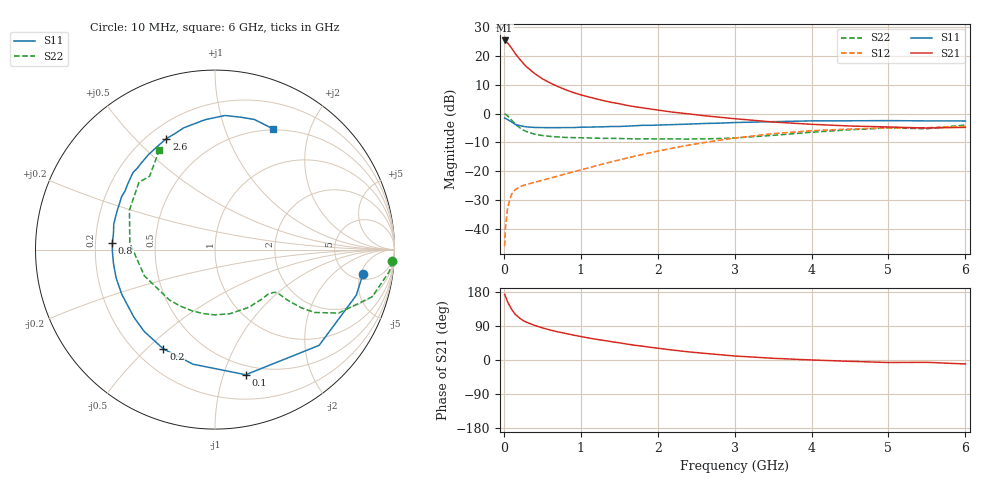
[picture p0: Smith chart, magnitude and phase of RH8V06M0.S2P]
! SIEMENS Small Signal Semiconductors
! BFR106
! Si NPN RF Bipolar Junction Transistor in SOT23
! VCE = 8 V  IC = 6 mA
! Common Emitter S-Parameters:  August  1996
# GHz  S  MA  R  50
!  f  S11  S21  S12  S22
! GHz  MAG  ANG  MAG  ANG  MAG  ANG  MAG  ANG
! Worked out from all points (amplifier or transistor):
!   36 points, 10 MHz to 6 GHz, reference 50 ohm
!   highest |S21| = 25.4 dB at 10 MHz (marker M1)
!   |S21| within 3 dB of that: start of sweep to 109.4 MHz
!   unconditionally stable (mu >= 1): 589.9 MHz to 1.841 GHz; 5.092 GHz to end of sweep
!   at 250 MHz: K = 0.55, MSG = 21.2 dB, |S12| = -24.9 dB
!   at 1.4 GHz: K = 1.11, MAG = 8.3 dB, |S12| = -16.7 dB
!   at 6 GHz: K = 1.01, MAG = -0.9 dB, |S12| = -4.4 dB
!   S11 on the Smith chart (normalised r, x): 10 MHz: 6.22, -5.51; 100 MHz: 0.41, -1.19; 200 MHz: 0.31, -0.56; 800 MHz: 0.27, +0.03; 2.6 GHz: 0.27, +0.62; 6 GHz: 0.49, +1.48
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0.01  0.8357 -9.2  18.66 173.5  0.005 88.2  0.9907 -3.8
0.02  0.8275 -17.9  18.42 168.7  0.0101 82.7  0.9778 -7.3
0.05  0.7881 -42.6  16.81 152.9  0.0239 68.8  0.9142 -16.7
0.1  0.7179 -76.2  13.79 134.0  0.0398 55.2  0.7738 -27.2
0.15  0.6501 -100.9  10.98 120.0  0.0479 47.3  0.6555 -32.3
0.2  0.6234 -117.5  9.019 111.4  0.0531 44.1  0.5785 -34.0
0.25  0.6031 -130.8  7.531 104.1  0.0566 42.1  0.5209 -34.6
0.3  0.5883 -140.2  6.429 99.2  0.0592 42.4  0.4853 -34.9
0.4  0.5761 -154.5  4.98 91.4  0.0641 43.9  0.4402 -34.7
0.5  0.5729 -164.2  4.036 84.8  0.0697 46.4  0.417 -35.0
0.6  0.5709 -172.1  3.42 79.3  0.0756 49.2  0.4031 -36.3
0.8  0.5733 176.3  2.61 70.2  0.0897 54.7  0.3863 -40.1
0.9  0.5727 171.1  2.33 65.9  0.0972 57.2  0.3833 -42.1
1.1  0.5838 161.4  1.952 58.2  0.1143 60.6  0.3783 -48.1
1.6  0.6073 143.5  1.392 42.0  0.1692 64.6  0.3678 -64.9
2.2  0.6456 125.2  1.06 26.1  0.253 61.8  0.3634 -90.3
2.6  0.6746 113.7  0.922 17.7  0.314 56.7  0.3642 -110.6
3.5  0.726 94.3  0.716 4.5  0.4492 41.2  0.4199 -159.7
4.5  0.7515 79.0  0.61 -3.5  0.5406 21.4  0.5252 155.2
5  0.7576 73.2  0.587 -6.6  0.564 13.1  0.5658 138.5
5.5  0.7482 67.5  0.562 -6.1  0.5692 8.6  0.5473 131.8
6  0.7459 64.1  0.578 -10.5  0.6047 0.4  0.6353 119.2
